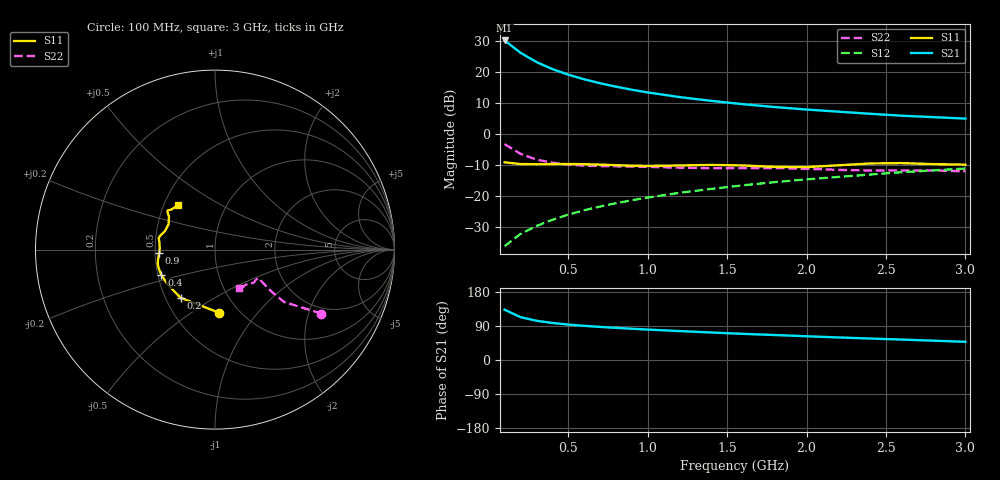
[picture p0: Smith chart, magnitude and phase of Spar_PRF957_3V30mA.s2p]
! Filename:  PRF957H.S2P  Version:  3.0
! NXP part #:  PRF957  Date:  Nov 1998
! Bias condition:  Vce=3V, Ic=30mA
#  MHz  S  MA  R 50
! Freq  S11  S21  S12  S22
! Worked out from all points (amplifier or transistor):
!   20 points, 100 MHz to 3 GHz, reference 50 ohm
!   highest |S21| = 30.3 dB at 100 MHz (marker M1)
!   |S21| within 3 dB of that: start of sweep to 175.2 MHz
!   unconditionally stable (mu >= 1): 567.7 MHz to end of sweep
!   at 400 MHz: K = 0.95, MSG = 24.4 dB, |S12| = -27.6 dB
!   at 1.2 GHz: K = 1.05, MAG = 14.1 dB, |S12| = -18.9 dB
!   at 3 GHz: K = 1.03, MAG = 7.0 dB, |S12| = -11.1 dB
!   S11 on the Smith chart (normalised r, x): 100 MHz: 0.81, -0.65; 200 MHz: 0.60, -0.36; 400 MHz: 0.52, -0.17; 900 MHz: 0.53, -0.02; 3 GHz: 0.59, +0.32
100  0.3524 -86.2  32.8 132.7  0.01556 69.1  0.6921 -31.0
200  0.3301 -125.6  20.73 113.1  0.02454 68.5  0.4831 -37.2
300  0.3281 -144.3  14.71 103.6  0.0329 70.9  0.391 -36.6
400  0.3304 -154.6  11.32 97.7  0.04149 73.1  0.3465 -35.5
500  0.3309 -161.1  9.192 93.5  0.0503 74.7  0.3237 -34.6
600  0.3288 -165.6  7.741 90.2  0.05911 75.8  0.3121 -34.2
700  0.3235 -169.4  6.682 87.3  0.06804 76.4  0.3067 -33.8
800  0.3168 -173.1  5.882 84.8  0.07687 76.9  0.3037 -33.4
900  0.311 -177.0  5.248 82.5  0.08587 77.3  0.3009 -33.1
1000  0.3081 178.9  4.744 80.3  0.09493 77.4  0.2979 -32.9
1200  0.313 172.1  3.991 76.4  0.1132 77.3  0.2886 -33.8
1400  0.3203 168.2  3.469 72.6  0.131 76.8  0.2827 -36.5
1600  0.3135 165.3  3.065 69.0  0.1497 76.4  0.2834 -39.2
1800  0.2974 159.9  2.754 65.9  0.1686 75.6  0.2837 -40.8
2000  0.2947 151.4  2.51 62.7  0.1868 75.0  0.2771 -42.2
2200  0.3153 144.4  2.319 59.5  0.2045 74.2  0.2658 -45.2
2400  0.3376 141.7  2.145 56.7  0.2235 73.2  0.2598 -49.7
2600  0.3419 140.4  1.995 53.9  0.2442 72.0  0.2611 -53.7
2800  0.3293 137.1  1.89 50.9  0.2612 71.3  0.2605 -56.1
3000  0.323 130.1  1.794 48.0  0.2798 70.6  0.2522 -58.4
